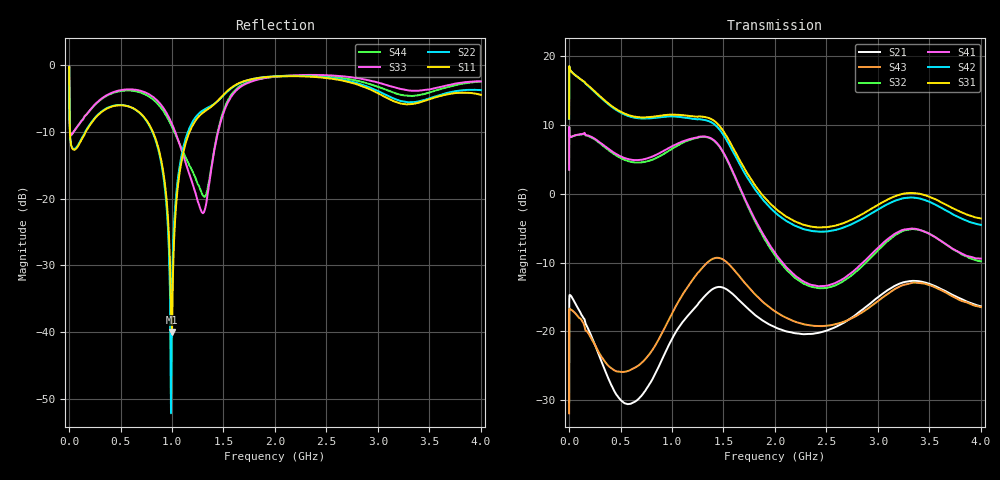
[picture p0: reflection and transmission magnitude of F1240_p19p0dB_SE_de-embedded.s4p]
! Integrated Device Technology
! Corporate Headquarters
! 6024 Silver Creek Valley Road
! San Jose, CA 95138  USA
! Phone:  1-408-284-8200
! Toll Free:  1-800-223-1366
! Webpage:  http://www.idt.com/
! Timing and RF Division
! 515 Groton Road, Suite 102
! Westford, MA 01886-6024
! Device:  F1240
! Description: Dual Intermediate Frequency Digital Variable Gain Amplifier
! Frequency:  10.0 -  500.00 MHz
! Package:  5x5 mm QFN Plastic Package: 32 pin
! Ports:  8 RF, 20 DC
!  Pin  1  = GA3 / Data  Pin 17  = RF OUT_B+
!  Pin  2  = GA4 / CLK  Pin 18  = RF OUT_B-
!  Pin  3  = GA5  Pin 19  = STBY_B
!  Pin  4  = VMODE  Pin 20  = Ground
!  Pin  5  = No Connect  Pin 21  = Ground
!  Pin  6  = GB5  Pin 22  = STB_A
!  Pin  7  = GB4  Pin 23  = RF OUT_A-  = Port 4
!  Pin  8  = GB3  Pin 24  = RF OUT_A+  = Port 3
!  Pin  9  = GB2  Pin 25  = GA0
!  Pin 10  = GB1  Pin 26  = ISET_A
!  Pin 11  = RF IN_B+  Pin 27  = VCC
!  Pin 12  = RF IN_B-  Pin 28  = Ground
!  Pin 13  = Ground  Pin 29  = RF IN_A-  = Port 2
!  Pin 14  = VCC  Pin 30  = RF IN_A+  = Port 1
!  Pin 15  = ISET_B  Pin 31  = GA1
!  Pin 16  = GB0  Pin 32  = GA2 / CSb
! Gain  = +19.5 dB
! State  = 1
! Voltage  = +5.00 V
! Current  = 85.292 mA (one channel only)
! Temperture  =  +25 C
! Test Date  =  2017-10-18
! Board  =  EB4031
! Data:  The device was measured on a custom evaluation board which has
!  individual transmission lines to the RF pins.  Data was collected
!  using a calibrated network analyzer.  The evaluation board was
!  de-embedded using Automatic Fixture Removal.
!  The reference plane is the edge of the package pin.
!  Only Channel A was measured.
!  This data is in single-ended operation.  If your needs are balanced
!  or differential S-parameters then this file needs to be used a
!  linear simulator.
! File Date:  2017-11-10  MJV
! Note:
!  Integrated Device Technology supplies this data as a sample of measured
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# Hz S dB R 100
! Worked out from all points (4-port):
!   410 points, 500 kHz to 4 GHz, reference 100 ohm
!   strongest paths, dB at 500 kHz, 930 MHz, 1.96 GHz, 2.98 GHz, 4 GHz:
!     S31: 10.9, 11.5, -1.5, -1.8, -3.6
!     S42: 10.9, 11.2, -2.1, -2.5, -4.5
!     S41: 3.5, 6.3, -7.7, -8.2, -9.4
!     S32: 3.5, 5.9, -8.1, -8.5, -9.8
!     S43: -31.9, -19.5, -16.7, -15.8, -16.5
!     S21: -30.3, -23.2, -19.1, -15.3, -16.4
!   lowest |S11| = -40.0 dB at 1 GHz (marker M1), VSWR 1.02, Z = 99.3 - j1.87 ohm
!   |S11| at or under -10 dB: 8.467 MHz to 160.4 MHz (151.9 MHz wide, 180 % of centre); 814.6 MHz to 1.17 GHz (355.3 MHz wide, 35.8 % of centre)
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500000  -0.31 -6.8  -30.11 27.0  -27.67 69.4  -63.68 66.8
        -30.30 26.3  -0.30 -6.7  -63.56 65.7  -27.67 70.6
        10.93 -105.6  3.50 72.5  -0.43 0.6  -31.97 -176.2
        3.50 73.6  10.91 -104.4  -31.93 -176.5  -0.44 2.9
4000000  -7.08 -44.6  -14.81 12.9  -22.02 5.0  -39.75 35.8
         -14.82 12.8  -7.06 -44.6  -39.77 35.9  -22.03 5.0
         18.32 -172.0  8.55 1.3  -6.71 -38.5  -16.75 22.0
         8.53 1.2  18.30 -171.8  -16.72 21.9  -6.77 -38.4
2.1e8  -8.80 -107.6  -20.45 -116.3  -24.79 -52.6  -33.11 9.9
       -20.46 -115.1  -8.69 -109.4  -33.17 10.1  -24.80 -52.4
       15.44 105.9  8.25 -62.6  -6.59 -78.5  -20.31 -127.1
       8.34 -62.5  15.38 105.0  -20.89 -126.2  -6.61 -77.9
5.6e8  -6.09 -171.2  -29.94 87.0  -26.42 -106.6  -27.37 -60.8
       -30.57 84.9  -6.08 -172.5  -27.55 -59.7  -26.59 -107.0
       11.55 19.8  4.82 -146.5  -3.61 -150.7  -25.09 87.0
       5.11 -147.5  11.41 18.6  -25.83 67.0  -3.78 -150.2
1e9  -40.00 -109.5  -19.42 -31.7  -23.10 162.5  -22.33 -164.3
     -21.10 -31.3  -33.05 -76.4  -22.70 -160.2  -23.55 162.0
     11.53 -85.1  6.55 120.1  -8.81 147.1  -16.09 -10.5
     6.91 115.0  11.26 -86.9  -17.41 -31.1  -9.22 153.4
1.5e9  -4.40 -135.4  -13.72 164.9  -31.29 47.3  -23.51 67.1
       -13.67 170.1  -4.51 -137.0  -23.59 73.2  -33.64 39.9
       9.09 117.2  5.91 -58.7  -7.12 -105.1  -9.20 165.0
       5.99 -63.8  8.55 115.7  -9.59 158.0  -6.78 -109.1
4e9  -4.41 -159.1  -16.40 52.6  -22.10 -31.0  -19.13 -48.1
     -16.37 52.0  -3.72 -152.0  -21.81 -29.6  -25.88 -10.0
     -3.59 -3.5  -9.83 -145.7  -2.41 -135.3  -14.47 89.8
     -9.44 -155.6  -4.51 5.3  -16.48 63.3  -2.43 -140.0
